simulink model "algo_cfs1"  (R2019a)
settings: configuration reference "configurationSettings" (kept in a data dictionary, not in this file)
undefined symbols (not defined in the file or in its folder): algo_cfs1_fp, algo_cfs1_tp, DiscIntNeverNeededParam, ProductionState, QualityTag, signal1, signal2, signal3, Value

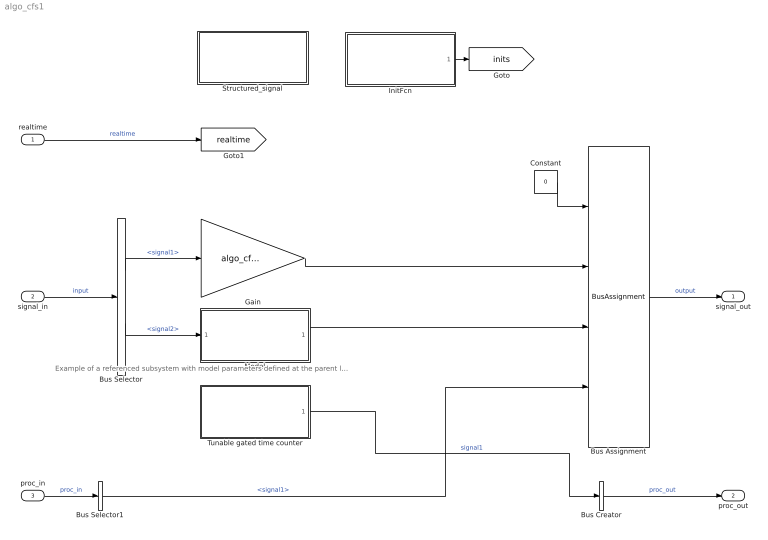
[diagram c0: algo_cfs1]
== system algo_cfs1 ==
  note: Example of a referenced subsystem with model parameters defined at the parent level
  realtime : Inport  OutDataTypeStr=single  PortDimensions=1  SampleTime=algo_cfs1_fp.timing.dt  Interpolate=off
  signal_in : Inport  Port=2  OutDataTypeStr=Bus: algo_cfs1_inBus  PortDimensions=1  Interpolate=off
  proc_in : Inport  Port=3  OutDataTypeStr=Bus: algo_cfs2_procout  PortDimensions=1  SampleTime=algo_cfs1_fp.timing.dt  Interpolate=off
  Bus Assignment : BusAssignment  AssignedSignals=signal1,signal2,signal3
  Bus Creator : BusCreator  Inputs=1
  Bus Selector : BusSelector  OutputSignals=signal1,signal2
  Bus Selector1 : BusSelector  OutputSignals=signal1
  Constant : Constant  Value=0  OutDataTypeStr=Bus: algo_cfs1_outBus
  Gain : Gain  Gain=algo_cfs1_tp.gain
  InitFcn : Subsystem  TreatAsAtomicUnit=on
  Model : ModelReference  ModelNameDialog=algo_cfs1_referenced.slx  ParameterArgumentNames=TP  ParameterArgumentValues=algo_cfs1_tp.refmodel  UsingDefaultArgumentValue=0  SimulationMode=Normal  ModelReferenceVersion=1.15
  Structured_signal : Subsystem  Commented=on
  Tunable gated time counter : Subsystem
  signal_out : Outport  OutDataTypeStr=Bus: algo_cfs1_outBus
  proc_out : Outport  Port=2  OutDataTypeStr=Bus: algo_cfs1_procout
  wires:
  signal_in/1 -> Bus Selector/1  "input"
  Bus Selector/1 -> Gain/1  "<signal1>"
  Constant/1 -> Bus Assignment/1
  realtime/1 -> [realtime]  "realtime"
  Bus Assignment/1 -> signal_out/1  "output"
  Model/1 -> Bus Assignment/3
  Bus Selector/2 -> Model/1  "<signal2>"
  InitFcn/1(InitOut) -> [inits]
  Gain/1 -> Bus Assignment/2
  Bus Creator/1 -> proc_out/1  "proc_out"
  proc_in/1 -> Bus Selector1/1  "proc_in"
  Bus Selector1/1 -> Bus Assignment/4  "<signal1>"
  Tunable gated time counter/1(time) -> Bus Creator/1  "signal1"

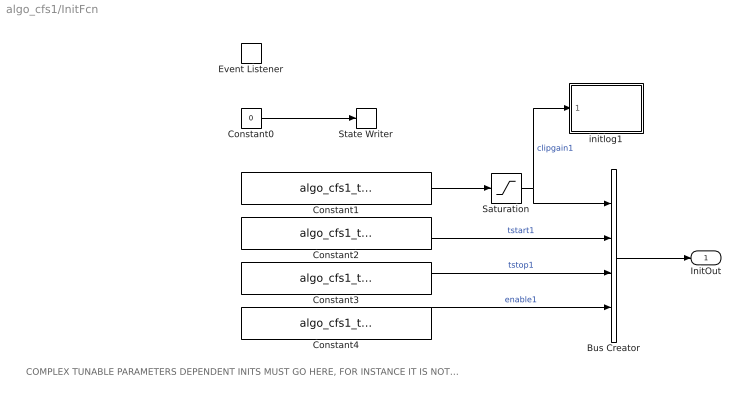
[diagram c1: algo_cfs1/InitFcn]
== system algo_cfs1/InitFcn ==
  note: COMPLEX TUNABLE PARAMETERS DEPENDENT INITS MUST GO HERE, FOR INSTANCE IT IS NOT POSSIBLE TO REFER TO A TUNABLE PARAMETER VIA DIRECT INDEXING IN MODEL DIALOG, THE VALUE MUST BE EXTRACTED HERE
  Bus Creator : BusCreator  Inputs=4
  Constant0 : Constant  Commented=on  Value=0
  Constant1 : Constant  Value=algo_cfs1_tp.gain  OutDataTypeStr=single
  Constant2 : Constant  Value=algo_cfs1_tp.colvect(1)  OutDataTypeStr=single
  Constant3 : Constant  Value=algo_cfs1_tp.colvect(2)  OutDataTypeStr=single
  Constant4 : Constant  Value=algo_cfs1_tp.enable  OutDataTypeStr=boolean
  Event Listener : EventListener  DisableCoverage=on  EventName=reset
  Saturation : Saturate
  State Writer : StateWriter  Commented=on
  initlog1 : MATLAB Function  TreatAsAtomicUnit=on
  InitOut : Outport  OutDataTypeStr=Bus: algo_cfs1_init1
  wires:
  Constant0/1 -> State Writer/1
  Bus Creator/1 -> InitOut/1
  Constant1/1 -> Saturation/1
  Constant2/1 -> Bus Creator/2  "tstart1"
  Saturation/1 -> initlog1/1(u), Bus Creator/1  "clipgain1"
  Constant3/1 -> Bus Creator/3  "tstop1"
  Constant4/1 -> Bus Creator/4  "enable1"

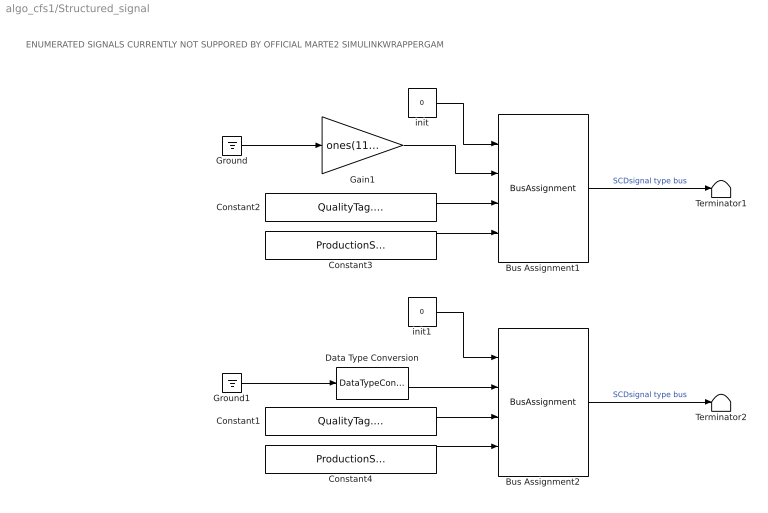
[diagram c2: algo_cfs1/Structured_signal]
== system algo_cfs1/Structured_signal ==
  note: ENUMERATED SIGNALS CURRENTLY NOT SUPPORED BY OFFICIAL MARTE2 SIMULINKWRAPPERGAM
  Bus Assignment1 : BusAssignment  AssignedSignals=Value,QualityTag,ProductionState
  Bus Assignment2 : BusAssignment  AssignedSignals=Value,QualityTag,ProductionState
  Constant1 : Constant  Value=QualityTag.INVALID  OutDataTypeStr=Enum: QualityTag
  Constant2 : Constant  Value=QualityTag.GOOD  OutDataTypeStr=Enum: QualityTag
  Constant3 : Constant  Value=ProductionState.RUNNING  OutDataTypeStr=Enum: ProductionState
  Constant4 : Constant  Value=ProductionState.OUTDATED  OutDataTypeStr=Enum: ProductionState
  Data Type Conversion : DataTypeConversion  OutDataTypeStr=int32
  Gain1 : Gain  Gain=ones(11,1)
  Ground : Ground
  Ground1 : Ground
  Terminator1 : Terminator
  Terminator2 : Terminator
  init : Constant  Value=0  OutDataTypeStr=Bus: SCDBus_single_11_Vector
  init1 : Constant  Value=0  OutDataTypeStr=Bus: SCDBus_int32_Scalar
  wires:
  Constant4/1 -> Bus Assignment2/4
  Data Type Conversion/1 -> Bus Assignment2/2
  Ground/1 -> Gain1/1
  Constant1/1 -> Bus Assignment2/3
  init1/1 -> Bus Assignment2/1
  init/1 -> Bus Assignment1/1
  Bus Assignment1/1 -> Terminator1/1  "SCDsignal type bus"
  Bus Assignment2/1 -> Terminator2/1  "SCDsignal type bus"
  Constant2/1 -> Bus Assignment1/3
  Constant3/1 -> Bus Assignment1/4
  Gain1/1 -> Bus Assignment1/2
  Ground1/1 -> Data Type Conversion/1

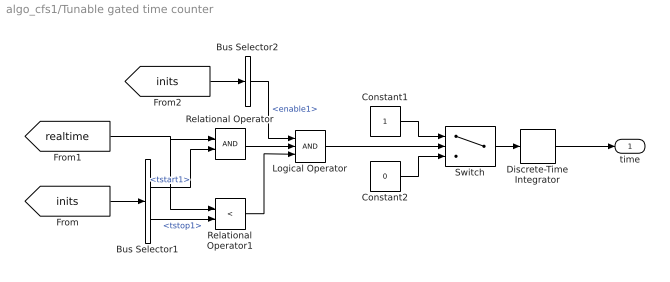
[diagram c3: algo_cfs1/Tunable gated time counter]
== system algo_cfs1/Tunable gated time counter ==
  Bus Selector1 : BusSelector  OutputSignals=tstart1,tstop1
  Bus Selector2 : BusSelector  OutputSignals=enable1
  Constant1 : Constant  OutDataTypeStr=single
  Constant2 : Constant  Value=0  OutDataTypeStr=single
  Discrete-Time Integrator : DiscreteIntegrator  SampleTime=-1  ICPrevOutput=DiscIntNeverNeededParam  ICPrevScaledInput=DiscIntNeverNeededParam
  Logical Operator : Logic  Inputs=3  AllPortsSameDT=off  OutDataTypeStr=boolean
  Relational Operator : RelationalOperator  OutDataTypeStr=boolean  RndMeth=Simplest
  Relational Operator1 : RelationalOperator  Operator=<  OutDataTypeStr=boolean  RndMeth=Simplest
  Switch : Switch  Criteria=u2 > Threshold
  time : Outport
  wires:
  Bus Selector1/2 -> Relational Operator1/2  "<tstop1>"
  Discrete-Time Integrator/1 -> time/1
  Relational Operator1/1 -> Logical Operator/3
  Bus Selector2/1 -> Logical Operator/1  "<enable1>"
  [inits] -> Bus Selector1/1
  [realtime] -> Relational Operator1/1, Relational Operator/1
  Bus Selector1/1 -> Relational Operator/2  "<tstart1>"
  [inits] -> Bus Selector2/1
  Relational Operator/1 -> Logical Operator/2
  Constant1/1 -> Switch/1
  Constant2/1 -> Switch/3
  Switch/1 -> Discrete-Time Integrator/1
  Logical Operator/1 -> Switch/2

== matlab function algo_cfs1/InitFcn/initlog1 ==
function fcn(u)

fprintf('par value is %f\n',u);
